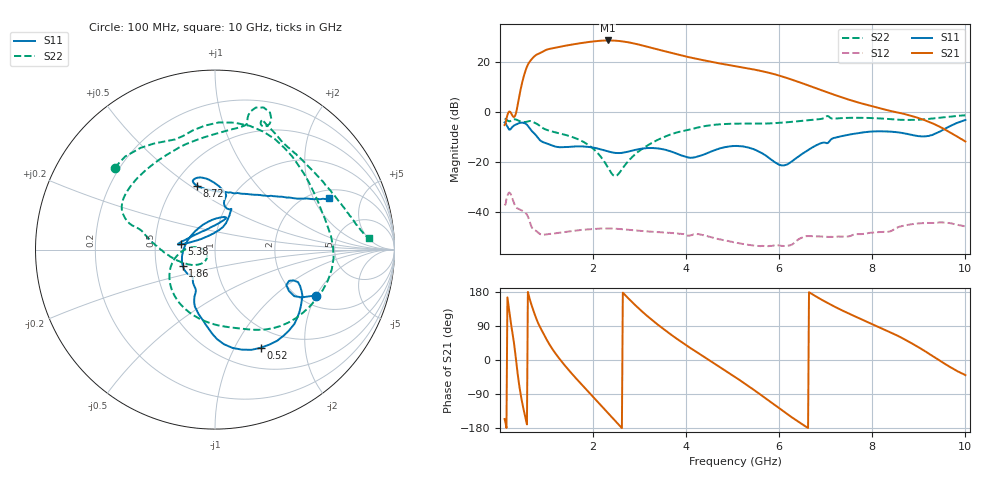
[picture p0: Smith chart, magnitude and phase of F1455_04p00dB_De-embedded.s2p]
! Integrated Device Technology
! Corporate Headquarters
! 6024 Silver Creek Valley Road
! San Jose, CA 95138  USA
! Phone:  1-408-284-8200
! Toll Free:  1-800-223-1366
! Webpage:  http://www.idt.com/
! Timing and RF Division
! 515 Groton Road, Suite 102
! Westford, MA 01886-6024
! Device:  F1455
! Description: 6-bit 0.5 dB Transmit Variable Gain Amplifier
! Frequency:  1400.0 -  2300.00 MHz
! Package:  6x6 mm Thin QFN Plastic Package: 28 pin
! State:  8
! Atten State:  4.0 dB
! Voltage:  +5.00 Volts
! Current:  216.111 mA
! Data:  The device was measured on a the F1455 evaluation board which has
!  individual transmission lines to the RF pins.  Data was collected
!  using a calibrated network analyzer.  The evaluation board was
!  de-embedded using a TRL calibration technique.
!  The reference plane is the edge of the package pin.
!  Pin  1 = CSb
!  Pin  2 = DATA
!  Pin  3 = CLK
!  Pin  4 = RSET
!  Pin  5 = GND
!  Pin  6 = RFIN  = Port 1
!  Pin  7 = GND
!  Pin  8 = NC
!  Pin  9 = NC
!  Pin 10 = NC
!  Pin 11 = NC
!  Pin 12 = NC
!  Pin 13 = NC
!  Pin 14 = /STBY
!  Pin 15 = GND
!  Pin 16 = RFOUT  = Port 2
!  Pin 17 = GND
!  Pin 18 = NC
!  Pin 19 = NC
!  Pin 20 = NC
!  Pin 21 = GND
!  Pin 22 = NC
!  Pin 23 = GND
!  Pin 24 = NC
!  Pin 25 = NC
!  Pin 26 = NC
!  Pin 27 = GND
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# GHz S dB R 50
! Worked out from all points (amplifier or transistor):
!   496 points, 100 MHz to 10 GHz, reference 50 ohm
!   highest |S21| = 28.8 dB at 2.32 GHz (marker M1)
!   |S21| within 3 dB of that: 1.164 GHz to 3.264 GHz (2.1 GHz wide, 94.8 % of centre)
!   unconditionally stable (mu >= 1): start of sweep to end of sweep
!   at 1.74 GHz: K = 4.30, MAG = 28.3 dB, |S12| = -47.4 dB
!   at 5.06 GHz: K = 15.75, MAG = 20.5 dB, |S12| = -52.5 dB
!   at 10 GHz: K = 50.96, MAG = -3.0 dB, |S12| = -46.0 dB
!   S11 on the Smith chart (normalised r, x): 100 MHz: 2.41, -2.01; 520 MHz: 0.74, -1.28; 1.86 GHz: 0.69, -0.13; 5.38 GHz: 0.68, +0.04; 8.72 GHz: 0.65, +0.53; 10 GHz: 2.39, +2.64
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0.1  -4.14 -24.4  -5.20 -155.8  -37.47 41.1  -2.83 140.8
0.4  -4.51 -39.7  4.82 -55.0  -38.92 -113.2  -3.43 50.4
0.52  -4.39 -65.1  14.94 -137.5  -40.08 -152.3  -3.98 23.7
0.7  -7.89 -99.1  21.67 137.0  -46.80 153.9  -3.86 -20.7
0.82  -10.45 -112.6  23.40 97.4  -48.47 138.1  -5.03 -49.5
0.96  -12.32 -116.8  24.74 63.9  -49.25 123.9  -6.81 -73.7
1.14  -13.57 -126.2  25.71 26.5  -48.82 100.8  -7.90 -97.8
1.34  -14.10 -130.7  26.46 -6.3  -48.33 78.8  -8.83 -121.2
1.76  -13.77 -146.9  27.80 -65.3  -47.33 43.4  -11.62 -159.3
1.86  -13.89 -152.6  28.07 -78.6  -47.15 36.0  -12.71 -167.1
2.08  -14.56 -168.9  28.57 -107.7  -46.88 21.1  -16.08 178.2
2.32  -15.80 164.3  28.81 -139.9  -46.77 5.6  -22.30 174.8
2.6  -16.42 122.8  28.51 -177.2  -47.06 -11.1  -23.53 -133.7
2.9  -15.22 88.2  27.51 145.5  -47.57 -25.6  -17.03 -142.4
3.4  -14.60 70.8  25.15 92.5  -48.27 -44.8  -11.09 -176.3
4.08  -18.36 110.8  21.98 32.6  -49.64 -67.8  -6.99 164.4
5.06  -13.59 171.8  18.46 -45.6  -52.45 -103.0  -4.63 148.4
5.38  -14.46 170.9  17.39 -72.3  -53.50 -107.4  -4.61 137.3
6.7  -14.32 67.2  10.22 174.4  -49.87 -139.2  -3.13 78.3
8.36  -7.80 107.0  0.60 74.5  -48.04 168.2  -2.78 62.1
8.72  -8.67 105.5  -0.92 52.5  -45.47 157.1  -3.12 49.6
10  -3.17 24.3  -11.80 -39.9  -46.00 82.1  -1.29 4.5
